(* Logix 5000 DataType export JVL_AXIS_MIS; software revision 33.00 *)

TYPE JVL_AXIS_MIS :   // Drive Data
STRUCT
   ActualMode : DINT;
   ActualPosition : REAL;   // P_IST
   ActualVelocity : REAL;   // V_IST(16)
   ActualTorque : REAL;   // ACTUAL_TORQUE
   AxisStatus : JVL_MIS_STATUS;
   AxisWarnings : JVL_MIS_Warnings;
   AxisError : JVL_MIS_Error;
   RequestedMode : DINT;
   RequestedPosition : DINT;   // P_SOLL
   RequestedVelocity : DINT;   // V_SOLL
   RequestedAcceleration : DINT;   // A_SOLL
   RequestedDeceleration : DINT;
   GeneralCommand : DINT;
   CommandTorque : REAL;   // Requested Torque, T_SOLL
   ZeroSearchVelocity : REAL;   // Homing velocity
   ZeroSearchPosition : REAL;   // Homing position
   ZeroSearchTorque : DINT;   // Homing torque setpoint threshold value
   ZeroSearchTThreshold : DINT;   // Threshold for torque zerosearch trigger, usually 20% lower than running torque
   TravelConst : REAL;   // Factor to multiply P_IST and P_SOLL for scaling
   VelConst : REAL;   // Factor to multiply V_SOLL and V_IST to get scaled velocity value
   HomingType : DINT;   // Holds the reqested homingtype
   LoadFactor : DINT;   // Inertia ratio motor/load
   Configured : DINT;
   MSG_OutValue : DINT;   // Used in exp. output message to the motor
   MSG_InValue : DINT;   // Used in Exp. output message, to get value from motor
   MSG_OutInstance : DINT;   // Registernumber
   MSG_InInstance : DINT;   // Registernummer
   V_SOLL_CountsPerSample : REAL;
   AOI_Type : DINT;   // MIS_Disable = 1, MIS_Home = 2, MIS_Jog = 3, MIS_Position = 4, MIS_Reset = 5, MIS_Stop = 6
   Position_AppType : REAL;   // Position depending on the Application type
   MSG_Out_Execute : BOOL;   // Enable MSG_Out
   MSG_In_Execute : BOOL;   // Enable MSG_In
   ErrorReset : BOOL;
   MSG_Out_Busy : BOOL;
   MSG_In_Busy : BOOL;
   MSG_Out_Done : BOOL;
   MSG_In_Done : BOOL;
END_STRUCT
END_TYPE

TYPE JVL_MIS_Error :
STRUCT
   GeneralError : BOOL;
   FollowingError : BOOL;
   OutputDriver : BOOL;
   PositionLimit : BOOL;
   LowBusVoltage : BOOL;
   OverVoltage : BOOL;
   TemperatureLimit : BOOL;
   Internal : BOOL;
   AbsoluteMultiturnEncoderPositionLost : BOOL;
   AbsoluteMultiturnEncoderSensorCounting : BOOL;
   AbsoluteMultiturnEncoderCommsFailed : BOOL;
   SSIEncoderCounting : BOOL;
   ClosedLoop : BOOL;
   ExternalMemory : BOOL;
   AbsoluteSingleturnEncoder : BOOL;
   H4InternalEncoderError : BOOL;
   ZeroSearchTimeout : BOOL;
   CVIUnstable : BOOL;
   MotorDriverOverload : BOOL;
   Reserved_19 : BOOL;
   Reserved_20 : BOOL;
   Reserved_21 : BOOL;
   Reserved_22 : BOOL;
   Reserved_23 : BOOL;
   Reserved_24 : BOOL;
   Reserved_25 : BOOL;
   Reserved_26 : BOOL;
   STO_Alarm : BOOL;
   Reserved_28 : BOOL;
   STO : BOOL;
   Reserved_30 : BOOL;
   Reserved_31 : BOOL;
END_STRUCT
END_TYPE

TYPE JVL_MIS_STATUS :   // STATUS JVL Stepper
STRUCT
   Reserved_0 : BOOL;
   AutoCorrectionActive : BOOL;
   InPhysicalPosition : BOOL;
   AtVelocity : BOOL;
   InPosition : BOOL;
   Accelerating : BOOL;
   Decelerating : BOOL;
   ZeroSearchDone : BOOL;
   PasswordLock : BOOL;
   MagneticEncoderError : BOOL;
   H3CalibrationDataPresent : BOOL;
   H3LinearisationTableRecorded : BOOL;
   GeneralError : BOOL;
   H3CalibrationDataLocked : BOOL;
   ElectromechBrakeActive : BOOL;
   ClosedLoopLeadLagDetected : BOOL;
   ClosedLoopActivated : BOOL;
   InternalEncoderCalibrated : BOOL;
   StandbyCurrentIsUsed : BOOL;
   STOEnabled : BOOL;
   InternalEncoderOK : BOOL;
   EthernetSyncActivated : BOOL;
   InTargetPosition : BOOL;
   STOChannelAOK : BOOL;
   STOChannelBOK : BOOL;
   External_memory_sizeA : BOOL;
   External_memory_sizeB : BOOL;
   Reserved_27 : BOOL;
   Reserved_28 : BOOL;
   Reserved_29 : BOOL;
   Reserved_30 : BOOL;
   Reserved_31 : BOOL;
END_STRUCT
END_TYPE

TYPE JVL_MIS_Warnings :
STRUCT
   PositiveLimitActive : BOOL;
   NegativeLimitActive : BOOL;
   PositiveLimitHasBeenReached : BOOL;
   NegativeLimitHasBeenReached : BOOL;
   LowBusVoltage : BOOL;
   Reserved_5 : BOOL;
   TemperatureWarning : BOOL;
   SSIEncoder : BOOL;
   DriverOverload : BOOL;
   STOActive : BOOL;
   Reserved_10 : BOOL;
   Reserved_11 : BOOL;
   Reserved_12 : BOOL;
   Reserved_13 : BOOL;
   Reserved_14 : BOOL;
   Reserved_15 : BOOL;
   Reserved_16 : BOOL;
   Reserved_17 : BOOL;
   Reserved_18 : BOOL;
   Reserved_19 : BOOL;
   Reserved_20 : BOOL;
   Reserved_21 : BOOL;
   Reserved_22 : BOOL;
   Reserved_23 : BOOL;
   Reserved_24 : BOOL;
   Reserved_25 : BOOL;
   Reserved_26 : BOOL;
   Reserved_27 : BOOL;
   Reserved_28 : BOOL;
   Reserved_29 : BOOL;
   Reserved_30 : BOOL;
   Reserved_31 : BOOL;
END_STRUCT
END_TYPE
